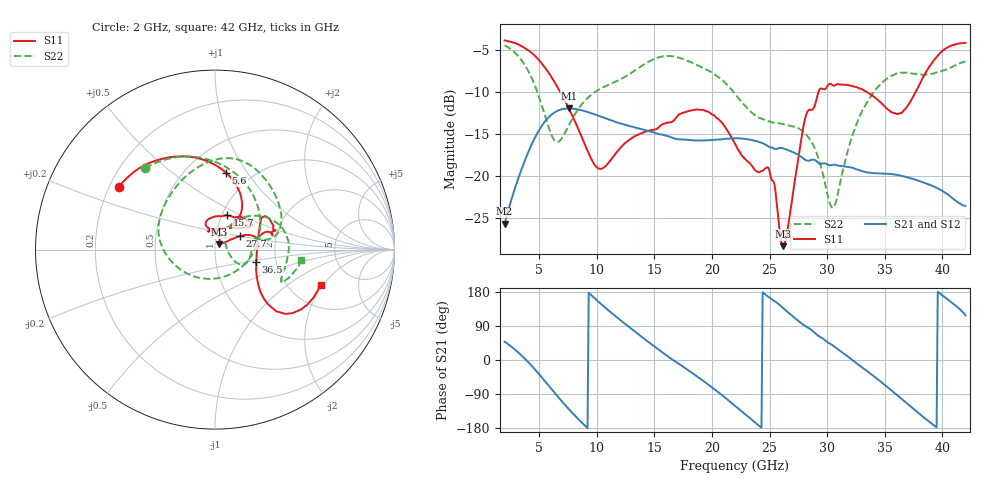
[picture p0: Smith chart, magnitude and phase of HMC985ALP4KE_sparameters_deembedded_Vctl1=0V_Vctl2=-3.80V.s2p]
!s2p File: Measurements: S11, S21, S12, S22
# GHz S dB R 50.0
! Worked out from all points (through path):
!   401 points, 2 GHz to 42 GHz, reference 50 ohm
!   highest |S21| = -11.97 dB at 7.6 GHz (marker M1); lowest = -25.7 dB at 2 GHz (marker M2)
!   lowest |S11| = -28.4 dB at 26.2 GHz (marker M3), VSWR 1.08, Z = 52.3 + j3.15 ohm
!   |S11| at or under -10 dB: 6.821 GHz to 29.25 GHz (22.43 GHz wide, 124 % of centre); 33.42 GHz to 37.69 GHz (4.271 GHz wide, 12 % of centre)
!   |S22| runs from -23.8 to -4.5 dB; largest |S21 - S12| = 0.00021
!   S11 on the Smith chart (normalised r, x): 2 GHz: 0.24, +0.28; 5.6 GHz: 0.76, +0.80; 15.7 GHz: 1.06, +0.42; 27.7 GHz: 1.30, +0.20; 36.5 GHz: 1.57, -0.23; 42 GHz: 2.95, -1.89
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2  -3.87 147.0  -25.72 48.5  -25.72 48.5  -4.46 130.7
3.6  -4.65 120.2  -18.76 8.1  -18.76 8.1  -6.49 85.3
4.6  -5.66 101.4  -15.55 -23.7  -15.55 -23.7  -9.15 48.4
5.6  -7.28 81.8  -13.37 -59.4  -13.37 -59.4  -13.26 -2.8
6.5  -9.22 66.4  -12.32 -92.4  -12.32 -92.4  -15.96 -69.2
7.6  -12.04 54.6  -11.97 -130.5  -11.98 -130.5  -13.92 -137.1
8.7  -15.40 54.9  -12.20 -165.1  -12.20 -165.1  -11.48 -171.3
10.4  -19.17 89.8  -12.97 147.0  -12.97 147.0  -9.56 161.4
15.4  -14.21 75.7  -15.04 26.8  -15.04 26.8  -5.87 86.0
15.7  -13.87 70.4  -15.11 20.1  -15.11 20.1  -5.78 82.2
19.2  -12.15 33.7  -15.79 -54.1  -15.79 -54.1  -7.12 37.0
22  -16.18 51.3  -15.53 -120.9  -15.53 -120.9  -10.24 10.9
24.9  -19.05 104.6  -16.51 166.6  -16.51 166.6  -13.49 12.8
26.2  -28.39 52.1  -16.75 136.3  -16.75 136.3  -13.87 -3.6
27.7  -16.12 28.6  -17.69 98.2  -17.69 98.1  -14.51 -24.1
28.7  -12.12 12.6  -18.08 77.6  -18.08 77.6  -16.08 -31.1
30.6  -9.26 19.6  -18.68 35.6  -18.67 35.6  -23.66 23.6
32.8  -9.58 34.0  -19.35 -14.2  -19.35 -14.3  -12.98 50.9
35.4  -12.22 11.7  -19.78 -75.7  -19.78 -75.7  -8.25 19.8
36.5  -12.47 -16.7  -20.02 -103.7  -20.03 -103.7  -7.71 6.1
39.5  -5.86 -43.6  -21.43 -177.8  -21.43 -177.8  -7.69 -25.6
42  -4.15 -18.5  -23.58 117.8  -23.59 117.7  -6.34 -6.7
